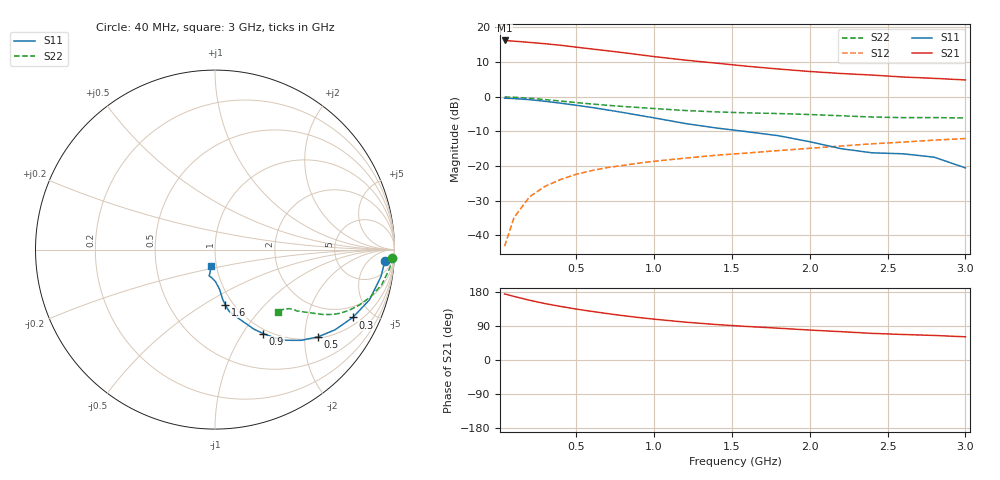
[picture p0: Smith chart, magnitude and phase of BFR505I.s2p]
! Filename:  BFR505I.S2P  Version:  3.0
! Philips part #: BFR505  Date: Feb 1992
! Bias condition: Vce=6V, Ic=2.5mA
#  MHz  S  MA  R  50
! Freq  S11  S21  S12  S22  !GUM [dB]
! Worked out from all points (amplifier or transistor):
!   21 points, 40 MHz to 3 GHz, reference 50 ohm
!   highest |S21| = 16.2 dB at 40 MHz (marker M1)
!   |S21| within 3 dB of that: start of sweep to 705.4 MHz
!   unconditionally stable (mu >= 1): 1.92 GHz to end of sweep
!   at 300 MHz: K = 0.29, MSG = 20.5 dB, |S12| = -25.8 dB
!   at 1 GHz: K = 0.71, MSG = 15.1 dB, |S12| = -18.6 dB
!   at 3 GHz: K = 1.08, MAG = 6.7 dB, |S12| = -12.1 dB
!   lowest NFmin = 1.30 dB at 900 MHz
!   S11 on the Smith chart (normalised r, x): 40 MHz: 15, -19; 300 MHz: 1.36, -3.84; 500 MHz: 1.04, -2.32; 900 MHz: 0.94, -1.24; 1.6 GHz: 0.92, -0.62; 3 GHz: 0.94, -0.17
40  0.949 -3.7  6.445 174.4  0.007 87.1  0.989 -2.6
100  0.937 -9.2  6.297 167.8  0.018 84.1  0.979 -6.1
200  0.905 -18.0  6.045 157.7  0.036 77.8  0.949 -12.0
300  0.856 -26.2  5.781 148.8  0.051 73.6  0.905 -16.9
400  0.804 -33.8  5.494 141.3  0.064 70.2  0.863 -20.9
500  0.751 -40.4  5.16 134.4  0.076 67.7  0.821 -24.3
600  0.698 -46.4  4.859 128.3  0.086 65.8  0.783 -26.9
700  0.643 -51.8  4.578 122.5  0.095 64.4  0.75 -28.8
800  0.591 -56.1  4.303 117.1  0.102 63.6  0.721 -30.1
900  0.54 -60.1  4.03 112.2  0.11 62.9  0.697 -31.2
1000  0.494 -63.9  3.775 107.8  0.117 62.4  0.673 -32.1
1200  0.41 -70.6  3.358 99.9  0.13 61.9  0.631 -33.8
1400  0.353 -77.1  3.036 93.6  0.143 62.1  0.602 -35.2
1600  0.312 -79.6  2.737 88.4  0.154 62.4  0.583 -36.0
1800  0.273 -81.5  2.498 83.9  0.167 63.3  0.57 -36.9
2000  0.224 -83.3  2.302 79.0  0.18 63.0  0.552 -37.2
2200  0.178 -89.2  2.154 74.8  0.194 63.0  0.53 -38.4
2400  0.155 -98.2  2.044 70.3  0.209 62.6  0.508 -40.6
2600  0.15 -102.6  1.915 67.3  0.221 62.8  0.498 -43.0
2800  0.134 -102.3  1.833 64.8  0.236 63.3  0.499 -44.4
3000  0.094 -102.7  1.739 61.2  0.249 63.0  0.492 -44.7
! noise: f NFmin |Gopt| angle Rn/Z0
900  1.3  0.631  16  0.74
2000  1.9  0.483  46  0.55
